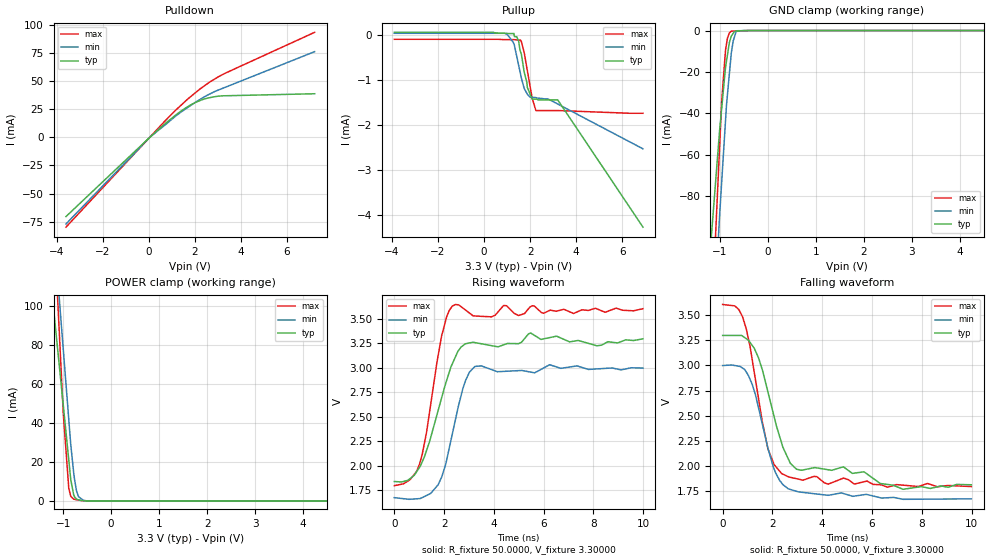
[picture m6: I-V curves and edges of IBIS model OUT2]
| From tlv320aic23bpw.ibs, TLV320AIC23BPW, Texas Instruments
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[Model] OUT2
Model_type Output
Vref=0.00000V
Rref=1.00000Gohms
Cref=10.0000pF
Vmeas=1.65000V
C_comp 2.00000pF 2.00000pF 2.00000pF
| variable typ   min   max
[Voltage Range] 3.30000V 3.00000V 3.60000V
[POWER Clamp Reference] 3.30000V 3.00000V 3.60000V
[Pullup Reference] 3.30000V 3.00000V 3.60000V
[Pulldown Reference] 0.00000V 0.00000V 0.00000V
[GND Clamp Reference] 0.00000V 0.00000V 0.00000V
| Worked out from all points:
|   slope of the pulldown table from 0 to 0.495 V, typ, clamps not added: 53.9 ohm
|   slope of the pullup table from 0 to 0.495 V, typ, clamps not added: 42.4 kohm
|   GND clamp passes 1 mA (typ) near -0.71 V on its own axis
|   POWER clamp passes 1 mA (typ) near -0.72 V on its own axis
|   falling waveform, R_fixture 50.0000, V_fixture 3.30000: 20-80 % time 1.03ns typ, 831ps min, 785ps max; typ from 3.3 V to 1.81 V
|   rising waveform, R_fixture 50.0000, V_fixture 3.30000: 20-80 % time 1.01ns typ, 728ps min, 689ps max; typ from 1.84 V to 3.3 V
[GND Clamp]
-3.6V     -819mA     -1.188A    -1.381A
-3V       -640.9mA   -934mA     -1.074A
-1.002V   -47.87mA   -88.79mA   -55.34mA
-961.9mV  -37.84mA   -73.69mA   -34.62mA
-880.9mV  -17.84mA   -43.59mA   -9.529mA
-840.7mV  -11.82mA   -31.07mA   -3.73mA
-800.3mV  -5.779mA   -20.9mA    -1.151mA
-759.8mV  -2.675mA   -10.71mA   -297.9uA
-719.4mV  -1.331mA   -4.956mA   -266.3uA
-658.7mV  -258.1uA   -412.8uA   -218.6uA
-494mV    -57.86uA   0A         -89.48uA
7.2V      0A         0A         0A
[Pulldown]
-3.6V     -70.56mA   -77.16mA   -80mA
61.43mV   526.4uA    546.8uA    613.8uA
1.199V    20.55mA    19.65mA    24.97mA
1.68V     27.36mA    26.6mA     34.07mA
2.039V    31.34mA    31.6mA     40.18mA
2.559V    35.09mA    37.91mA    48.2mA
3.161V    37.1mA     43.45mA    55.62mA
7.2V      38.97mA    76.52mA    93.74mA
[Pullup]
-3.9V     51.97uA    30.28uA    -102.6uA
891.1mV   30.73uA    30.28uA    -110.6uA
1.301V    25.82uA    -204.3uA   -110.7uA
1.499V    -143.5uA   -676.1uA   -119.3uA
1.621V    -437.4uA   -965.9uA   -155.6uA
1.742V    -831.6uA   -1.194mA   -400.4uA
1.858V    -1.062mA   -1.301mA   -737.1uA
1.878V    -1.169mA   -1.32mA    -795.9uA
2.088V    -1.428mA   -1.387mA   -1.407mA
2.25V     -1.428mA   -1.395mA   -1.682mA
3.198V    -1.447mA   -1.537mA   -1.682mA
6.9V      -4.267mA   -2.531mA   -1.742mA
[POWER Clamp]
-3.9V     762.4mA    988.7mA    1.509A
-1.282V   119.2mA    167.3mA    188.5mA
-1.201V   99.33mA    141.9mA    147.7mA
-1.12V    79.38mA    116.4mA    106.7mA
-1.079V   69.46mA    103.7mA    86.34mA
-998.4mV  49.61mA    78.38mA    45.6mA
-882.5mV  21.14mA    42.01mA    6.581mA
-842.1mV  11.21mA    29.34mA    2.489mA
-781.5mV  3.366mA    14.89mA    1.06mA
-680.3mV  640.8uA    2.303mA    525.5uA
-518.2mV  91.03uA    178.3uA    156.8uA
6.9V      0A         0A         0A
[Falling Waveform]
R_fixture = 50.0000
V_fixture = 3.30000
V_fixture_min = 3.00000
V_fixture_max = 3.60000
0s        3.297V     2.998V     3.605V
490ps     3.298V     2.999V     3.591V
800ps     3.291V     2.973V     3.483V
1.27ns    3.171V     2.747V     2.932V
1.82ns    2.736V     2.178V     2.17V
2.37ns    2.228V     1.832V     1.925V
2.97ns    1.968V     1.749V     1.874V
4.85ns    1.992V     1.727V     1.879V
7.25ns    1.769V     1.669V     1.81V
9.99ns    1.814V     1.674V     1.796V
[Rising Waveform]
R_fixture = 50.0000
V_fixture = 3.30000
V_fixture_min = 3.00000
V_fixture_max = 3.60000
0s        1.838V     1.674V     1.796V
1.01ns    1.982V     1.664V     2.013V
1.3ns     2.159V     1.697V     2.348V
1.76ns    2.563V     1.805V     3.124V
2.33ns    3.041V     2.323V     3.631V
2.76ns    3.228V     2.793V     3.611V
3.24ns    3.259V     3.015V     3.531V
4.39ns    3.236V     2.964V     3.638V
5.48ns    3.357V     2.957V     3.626V
9.99ns    3.297V     2.998V     3.605V
[Ramp]
| variable typ min max
dV/dt_r 875.398m/1.00576n 794.781m/718.406p 1.08543/689.195p
dV/dt_f 875.398m/977.721p 794.781m/832.344p 1.08543/788.764p
R_load = 50.0000Ohms
